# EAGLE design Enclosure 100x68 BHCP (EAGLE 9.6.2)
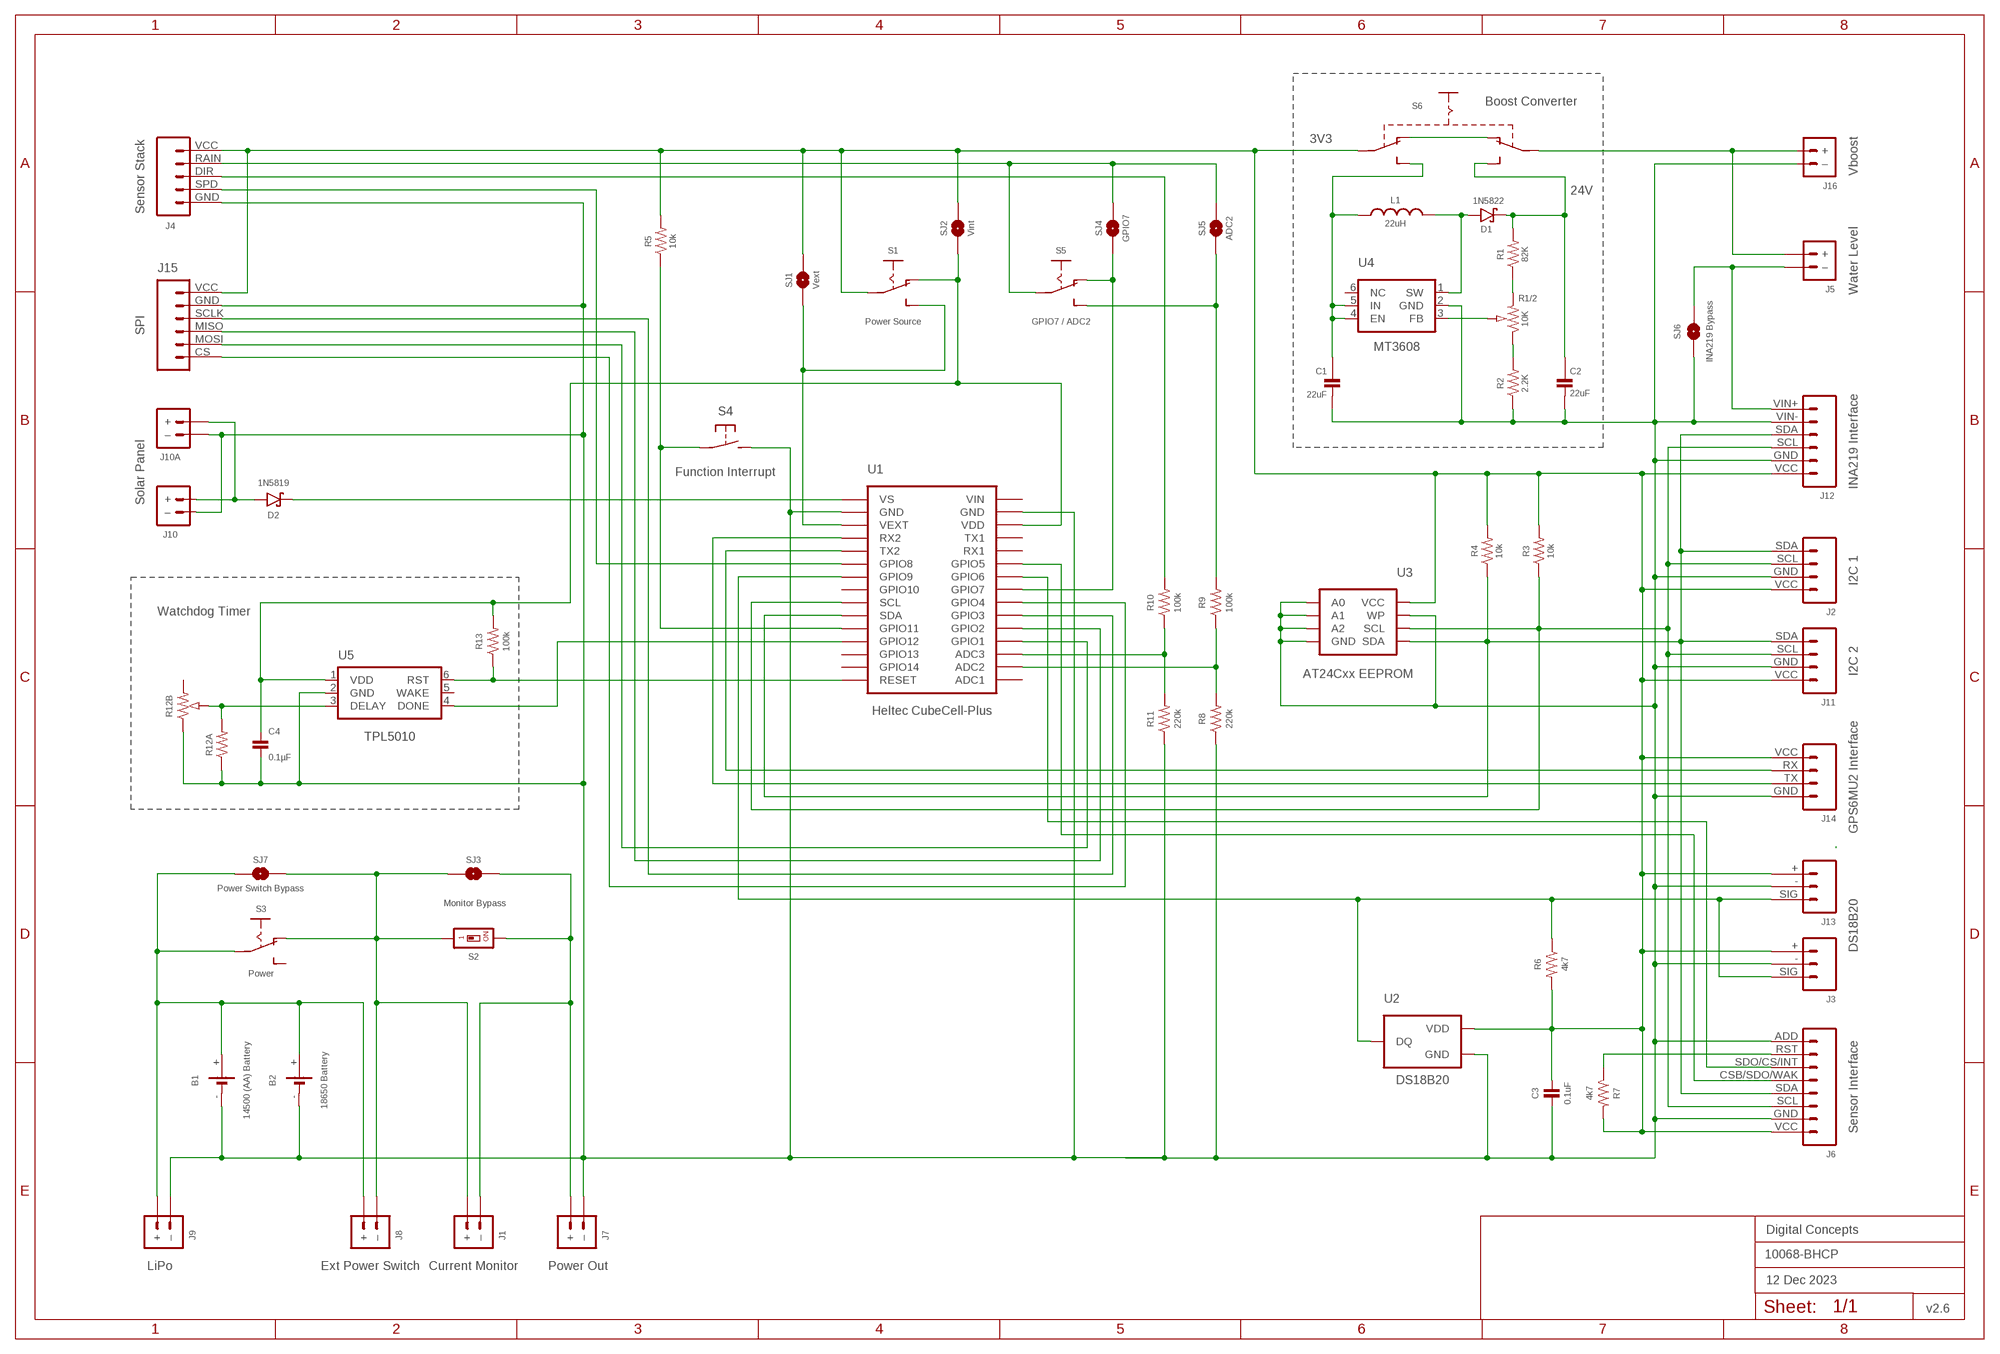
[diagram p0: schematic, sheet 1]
FRAME2 (A3L-LOC): DATE: 12 Dec 2023; OWNER: Digital Concepts; TITLE: 10068-BHCP; VERSION: v2.6

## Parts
B1  14500 (AA) Battery  BATTERY-HOLDER-14500(AA)  [BATTERY-14500]
B2  18650 Battery  BATTERY-HOLDER-18650  [BATTERY-18650]
C1  22uF  CAPACITOR-1206  [C1206]
C2  22uF  CAPACITOR-1206  [C1206]
C3  0.1uF  CAPACITOR-0805  [C0805]
C4  0.1µF  CAPACITOR-0805  [C0805]
D1  1N5822  DIODE-SCHOTTKY-1N5822  [DIODE_SMB]
D2  1N5819  1N5819-SOD-123  [SOD-123]
J1  Current Monitor  JST-PH2.0-2-HORIZONTALJST-PTH-2  [JST-PH2.0-2-HORIZONTAL]
J2  I2C 1  JST-PH2.0-4-VERTICAL-I2C  [JST-PH2.0-4-VERTICAL-I2C]
J3  DS18B20  JST-PH2.0-3-VERTICAL-DS18B20  [JST-PH2.0-3-VERTICAL-SIG]
J4  Sensor Stack  JST-PH2.0-5-DUAL-WEATHER  [JST-PH2.0-5-DUAL-WEATHER]
J5  Water Level  JST-PH2.0-2-DUAL-POWERJST-PTH-2  [JST-PH2.0-2-DUAL-POWER]
J6  Sensor Interface  HEADER-1X8-SENSOR  [CONN_08-SENSOR]
J7  Power Out  JST-GH1.25-2-HORIZONTAL-POWER  [JST-GH1.25-2-HORIZONTAL]
J8  Ext Power Switch  JST-PH2.0-2-DUAL-POWERJST-PTH-2  [JST-PH2.0-2-DUAL-POWER]
J9  LiPo  JST-PH2.0-2-HORIZONTAL-POWERJST-PTH-2  [JST-PH2.0-2-HORIZONTAL-POWER]
J10  Solar Panel  JST-PH2.0-2-VERTICAL  [JST-PH2.0-2-VERTICAL=POWER]
J10A  JST-PH2.0-2-HORIZONTAL-POWERJST-PTH-2  [JST-PH2.0-2-HORIZONTAL-POWER]
J11  I2C 2  JST-PH2.0-I2C-MALE-HORIZONTAL  [JST-PH2.0-4-HORIZONTAL]
J12  INA219 Interface  INA219-I2C-MODULE  [CONN_06-INA219]
J13  JST-PH2.0-3-HORIZONTAL-DS18B20  [JST-PH2.0-DS18B20-HORIZONTAL]
J14  GPS6MU2 Interface  HEADER-1X4-GPS  [CONN_04-GPS]
J15  SPI  JST-PH2.0-6-HORIZONTAL-SPI  [JST-PH2.0-6-HORIZONTAL-SPI]
J16  Vboost  JST-PH2.0-2-VERTICAL  [JST-PH2.0-2-VERTICAL=POWER]
L1  22uH  INDUCTOR-CDRH104R/6D28L5038P  [CDRH104R+6D28]
R1  82K  RESISTORR0805  [R0805]
R1/2  10K  RESISTOR-TRIMM-BAOTER-H-US  [RTRIM64P]
R2  2.2K  RESISTORR0805  [R0805]
R3  10k  RESISTORR0805  [R0805]
R4  10k  RESISTORR0805  [R0805]
R5  10k  RESISTORR0805  [R0805]
R6  4k7  RESISTORR0805  [R0805]
R7  4k7  RESISTORR0805  [R0805]
R8  220k  RESISTORR0805  [R0805]
R9  100k  RESISTORR0805  [R0805]
R10  100k  RESISTORR0805  [R0805]
R11  220k  RESISTORR0805  [R0805]
R12A  RESISTORR0805  [R0805]
R12B  RESISTOR-TRIMM-33-US  [RTRIM3*3]
R13  100k  RESISTORR0805  [R0805]
S1  Power Source  SWITCH-SLIDE-SPDT-SMT  [SWITCH-SPDT-SMT]
S2  Monitor Bypass  SWITCH-DIP-SWS001  [SMD-001]
S3  Power  SWITCH-SLIDE-SPDT-PTH  [SWITCH-SPDT-PTH]
S4  Function Interrupt  SWITCH-MOMENTARY-2-PIN  [SWITCH-2-PAD]
S5  GPIO7 / ADC2  SWITCH-SLIDE-SPDT-SMT  [SWITCH-SPDT-SMT]
S6  SWITCH-SLIDE-DPDT-PTH-S  [SWITCH-DPDT-PTH]
SJ1  Vext  SJ  [SJ]
SJ2  Vint  SJ-V-12  [SJ-VIA-12]
SJ3  Monitor  SJ  [SJ]
SJ4  GPIO7  SJ-V-2  [SJ-VIA-2]
SJ5  ADC2  SJ-V-12  [SJ-VIA-12]
SJ6  INA219 Bypass  SJ  [SJ]
SJ7  Power Switch Bypass  SJ  [SJ]
U1  Heltec CubeCell-Plus  HELTEC-CUBECELL-PLUS-X  [HELTEC-CUBECELL=PLUS-X]
U2  DS18B20  THERMOMETER-DS18B20  [TO-92]
U3  AT24Cxx EEPROM  AT24CXX-EEPROM  [SOP-8]
U4  MT3608  [SOT-23-6]
U5  TPL5010  TPL5010DDCR  [SOT-23-6]

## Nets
GND: B1.- B2.- C1.2 C2.2 C3.2 C4.2 J2.GND J3.- J4.GND J6.ADD J6.GND J7.-(–) J9.-(–) J10.-(–) J10A.-(–) J11.GND J12.GND J12.VIN- J13.- J14.GND J15.GND J16.-(–) R2.1 R8.1 R11.1 R12A.1 R12B.1(A) S4.P$2(S) SJ6.1 U1.GND@14(GND) U1.GND@17(GND) U2.1(GND) U3.P$1(A0) U3.P$2(A1) U3.P$3(A2) U3.P$4(GND) U3.P$7(WP) U4.2(GND) U5.2(GND)
N$1: D2.A J10.+ J10A.+
N$2: R10.1 R11.2 U1.ADC3
N$3: J1.2(–) J7.+ S2.2 SJ3.1
N$4: B1.+ B2.+ J8.+ J9.+ S3.2(P) SJ7.2
N$5: D2.C U1.VS
N$6: D1.A L1.1 U4.1(SW)
N$7: J4.DIR R10.2
N$8: J2.SCL J6.SCL J11.SCL J12.SCL R3.1 U1.SCL U3.P$6(SCL)
N$9: J6.RST R7.1
N$10: J6.CSB/SDO/WAK U1.GPIO5
N$11: J2.SDA J6.SDA J11.SDA J12.SDA R4.1 U1.SDA U3.P$5(SDA)
N$12: J4.SPD U1.GPIO8
N$13: S1.3(S) SJ1.1 U1.VEXT
N$14: J14.RX U1.TX2
N$15: J5.-(–) J12.VIN+ SJ6.2
N$16: J14.TX U1.RX2
N$18: R12A.2 R12B.2(S) U5.3(DELAY)
N$19: J6.SDO/CS/INT U1.GPIO6
N$20: J5.+ J16.+ S6.P$2(P1)
N$21: J1.1(+) J8.-(–) S2.1 S3.1(O) SJ3.2 SJ7.1
N$22: R1/2.2(S) U4.3(FB)
N$23: R1/2.1(A) R2.2
N$24: J3.SIG J13.SIG R6.1 U1.GPIO9 U2.2(DQ)
N$25: C1.1 L1.2 S6.P$6(S2) U4.4(EN) U4.5(IN)
N$26: S6.P$1(O1) S6.P$4(O2)
N$27: R5.1 S4.P$1(P) U1.GPIO11
N$28: C2.1 D1.C R1.2 S6.P$3(S1)
N$29: J15.MOSI U1.GPIO1
N$30: J15.MISO U1.GPIO2
N$31: R9.2 S5.3(S) SJ5.1 SJ5.1@V
N$32: J4.RAIN S5.2(P) SJ4.2 SJ4.2@V SJ5.2 SJ5.2@V
N$33: R8.2 R9.1 U1.ADC2
N$34: R13.1 U1.RST(RESET) U5.6(RST)
N$35: J15.SCLK U1.GPIO3
N$36: J15.CS U1.GPIO4
N$37: U1.GPIO12 U5.4(DONE)
N$38: R1.1 R1/2.3(E)
N$39: C4.1 R13.2 S1.1(O) SJ2.1 SJ2.1@V U1.VDD U5.1(VDD)
N$40: S5.1(O) SJ4.1 U1.GPIO7
VEXT: C3.1 J2.VCC J3.+ J4.VCC J6.VCC J11.VCC J12.VCC J13.+ J14.VCC J15.VCC R3.2 R4.2 R5.2 R6.2 R7.2 S1.2(P) S6.P$5(P2) SJ1.2 SJ2.2 SJ2.2@V U2.3(VDD) U3.P$8(VCC)
Unconnected: R12B.3(E) S3.3(S) U1.ADC1 U1.GPIO10 U1.GPIO13 U1.GPIO14 U1.RX1 U1.TX1 U4.6(NC) U5.5(WAKE)

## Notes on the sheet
- Boost Converter
- 3V3
- 24V
- Watchdog Timer

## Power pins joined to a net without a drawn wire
VIN: U1.VIN

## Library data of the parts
B1 = digitalconcepts:BATTERY-HOLDER-14500(AA): 14500 (AA) battery holder
B2 = digitalconcepts:BATTERY-HOLDER-18650: 18650 Battery Holder
C1 C2 = digitalconcepts:CAPACITOR-1206: 1206 Capacitor
C3 C4 = digitalconcepts:CAPACITOR-0805: 0805 Capacitor
D1 = digitalconcepts:DIODE-SCHOTTKY-1N5822: 1N5822 Schottky Diode SMB
D2 = digitalconcepts:1N5819-SOD-123: 1N5819 Schottky Diode SOD-123
J1 = digitalconcepts:JST-PH2.0-2-HORIZONTAL: PH2.0 2P Right Angle PCB Connector; PROD_ID: CONN-09863; SKU: PRT-09914
J2 = digitalconcepts:JST-PH2.0-4-VERTICAL-I2C: PH2.0 4P I2C Vertical Connector
J3 = digitalconcepts:JST-PH2.0-3-VERTICAL-DS18B20: DS18B20 PH2.0 Vertical PCB Connector
J4 = digitalconcepts:JST-PH2.0-5-DUAL-WEATHER: PH2.0 5P Dual Connector
J5 J8 = digitalconcepts:JST-PH2.0-2-DUAL-POWER: JST PH2.0 2P PTH Dual-Side Connector (Power); PROD_ID: CONN-09863; SKU: PRT-09914
J6 = digitalconcepts:HEADER-1X8-SENSOR: IoT Sensors 1x8 Pin Header for 'Sandwich' IoT Sensors
J7 = digitalconcepts:JST-GH1.25-2-HORIZONTAL-POWER: JST GH1.25 2P PTH Connector (Power)
J9 J10A = digitalconcepts:JST-PH2.0-2-HORIZONTAL-POWER: PH2.0 2P Right Angle PCB Connector; PROD_ID: CONN-09863; SKU: PRT-09914
J10 J16 = digitalconcepts:JST-PH2.0-2-VERTICAL: PH2.0 2P PCB Connector
J11 = digitalconcepts:JST-PH2.0-I2C-MALE-HORIZONTAL: PH2.0 4P (I2C) Right Angle PCB Connector
J12 = digitalconcepts:INA219-I2C-MODULE: INA219 I2C Module
J13 = digitalconcepts:JST-PH2.0-3-HORIZONTAL-DS18B20: DS18B20 PH2.0 Right Angle PCB Connector
J14 = digitalconcepts:HEADER-1X4-GPS: NEO GPS 4-Pin Header
J15 = digitalconcepts:JST-PH2.0-6-HORIZONTAL-SPI: PH2.0 6P Horizontal Connector—SPI
L1 = digitalconcepts:INDUCTOR-CDRH104R/6D28: Inductor; SPICEPREFIX: L
R1-R11 R12A R13 = digitalconcepts:RESISTOR: Resistor; SPICEPREFIX: R
R1/2 = digitalconcepts:RESISTOR-TRIMM-BAOTER-H-US: Trimm Resistor - Horizontal BAOTER
R12B = digitalconcepts:RESISTOR-TRIMM-3*3-US: Trimm Resistor - 3*3 SMD
S1 S5 = digitalconcepts:SWITCH-SLIDE-SPDT-SMT: Mini Sliding Switch SPDT SMT
S2 = digitalconcepts:SWITCH-DIP-SWS001: SMD Dip Switch 1 pol.
S3 = digitalconcepts:SWITCH-SLIDE-SPDT-PTH: Mini Sliding Switch SPDT PTH
S4 = digitalconcepts:SWITCH-MOMENTARY-2-PIN: 2 Pin Momentary Switch
S6 = digitalconcepts:SWITCH-SLIDE-DPDT-PTH-S: Switch DPDT PTH-S
SJ1 SJ3 SJ6 SJ7 = digitalconcepts:SJ: Solder Jumper
SJ2 SJ5 = digitalconcepts:SJ-V-12: Solder Jumper with Pad Vias
SJ4 = digitalconcepts:SJ-V-2: Solder Jumper with Pad Vias
U1 = digitalconcepts:HELTEC-CUBECELL-PLUS-X: Heltec CubeCell Dev-Board Plus Excluding internal pins
U2 = digitalconcepts:THERMOMETER-DS18B20: Digital Thermometer -55C-125C TO92-3; AVAILABILITY: Bad; DESCRIPTION: Temperature Sensor Digital, Local -55°C ~ 125°C 12 b 8-uMAX; MF: Maxim Integrated; MP: DS18B20; PACKAGE: TO-92 Maxim Integrated; PRICE: None
U3 = digitalconcepts:AT24CXX-EEPROM: AT24Cxx EEPROM SOP-8
U4 = digitalconcepts:MT3608: MT3608 DC-DC Step-Up Voltage Converter
U5 = digitalconcepts:TPL5010DDCR: TPL5010 Nano-Power System Timer with Watchdog

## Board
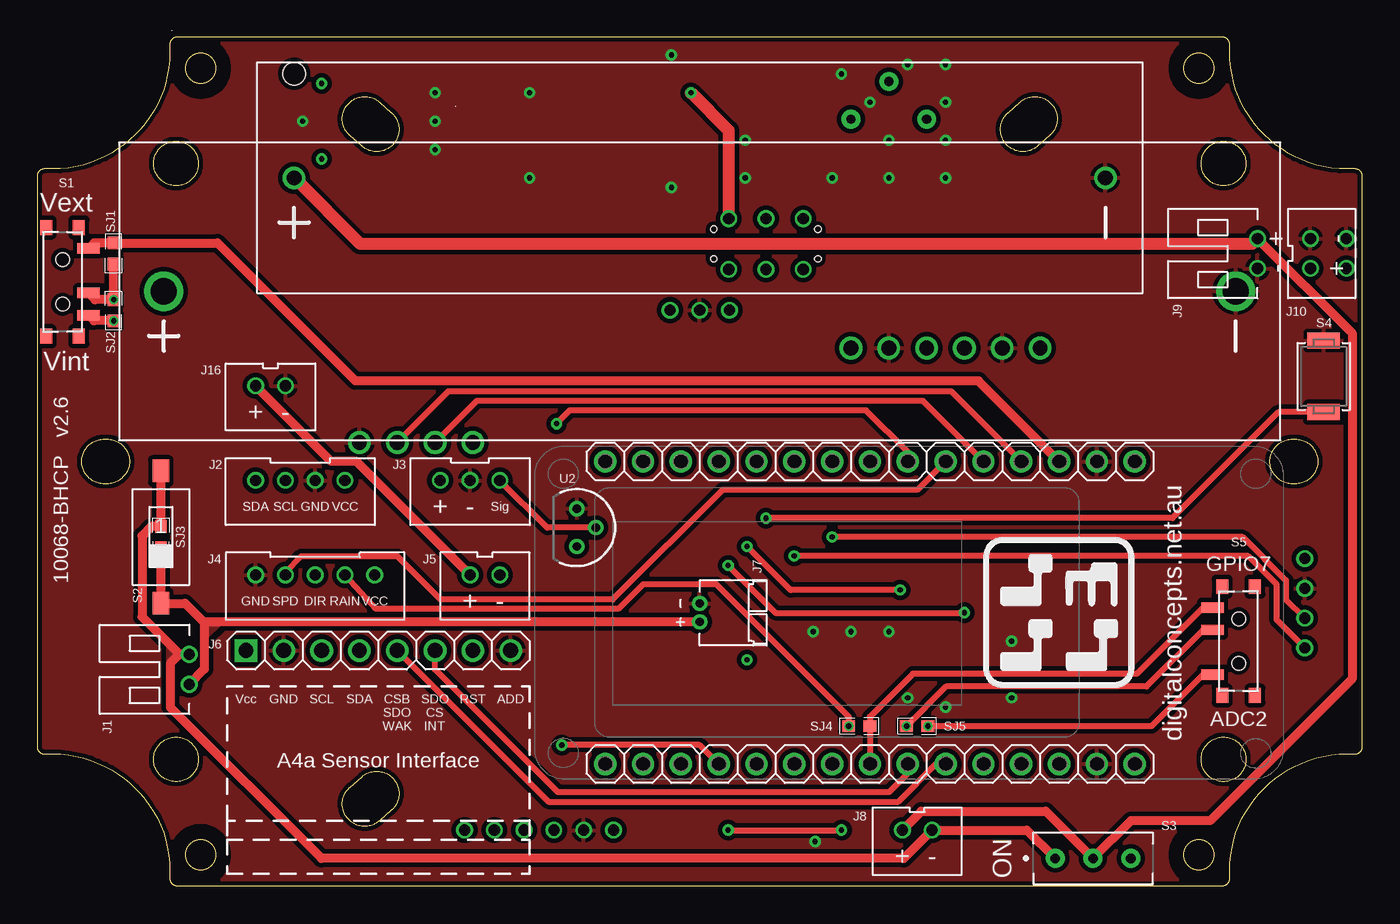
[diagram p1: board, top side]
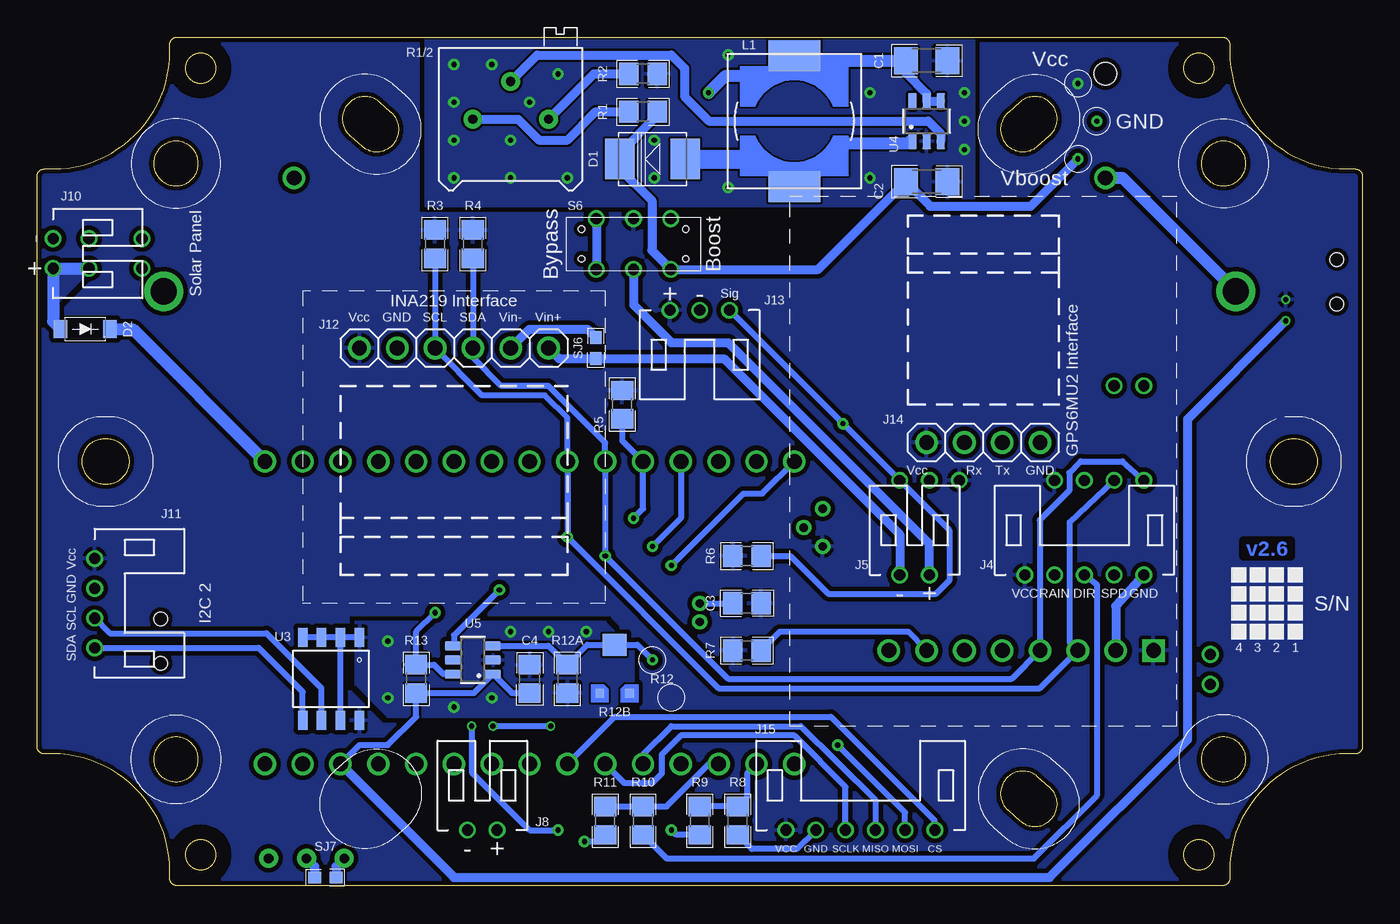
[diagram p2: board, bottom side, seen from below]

Size 89 x 57 mm. Coordinates in mm from the lower left corner, seen from the top.
Outline: 1134 segments
Outline: circle at 10.97,2.08 radius 1.02
Outline: circle at 10.97,54.92 radius 1.02
Outline: circle at 78.03,54.92 radius 1.02
Outline: circle at 78.03,2.08 radius 1.02
Copper layers (1*16): Top 0.035mm / dielectric 1.5mm / Bottom 0.035mm
Design rules "default *": minimum track width 6mil, minimum drill 0.35mm, track to track 6mil, track to pad 6mil, pad to pad 6mil, via to via 6mil, smd to smd 6mil, copper to edge 6mil, drill to drill 6mil, minimum pad ring 1mil, minimum via ring 8mil, stop-mask expansion 4mil, vias tented up to drill 0mil, thermal gap 10mil

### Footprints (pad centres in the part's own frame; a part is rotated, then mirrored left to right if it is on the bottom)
BATTERY-14500 = drill 1: + -27.25,0; - 27.25,0 | hole 1.524: -27.25,7
BATTERY-18650 = drill 1.75: + -36,0; - 36,0
C1206 = smd 1.6 x 1.8: 1 -1.4,0; 2 1.4,0
C0805 = smd 1.3 x 1.5: 1 -0.95,0; 2 0.95,0
DIODE_SMB = smd 2 x 2.7: A 2.2,0; C -2.2,0
SOD-123 = smd 0.91 x 1.22: A -1.65,0; C 1.65,0
JST-PH2.0-2-HORIZONTAL = drill 0.75: 1 1,0; 2 -1,0
JST-PH2.0-4-VERTICAL-I2C = drill 0.75: GND 1,0; SCL -1,0; SDA -3,0; VCC 3,0
JST-PH2.0-3-VERTICAL-SIG = drill 0.75: + -2,0; - 0,0; SIG 2,0
JST-PH2.0-5-DUAL-WEATHER = drill 0.75: DIR 0,0; GND 4,0; RAIN -2,0; SPD 2,0; VCC -4,0
JST-PH2.0-2-DUAL-POWER = drill 0.75: + 1,0; - -1,0
CONN_08-SENSOR = drill 1 pad 1.524: ADD 17.78,0; CSB/SDO/WAK 10.16,0; GND 2.54,0; RST 15.24,0; SCL 5.08,0; SDA 7.62,0; SDO/CS/INT 12.7,0 | drill 1 pad 1.524 square: VCC 0,0
JST-GH1.25-2-HORIZONTAL = drill 0.55 pad 1.016: + -0.625,0; - 0.625,0
JST-PH2.0-2-HORIZONTAL-POWER = drill 0.75: + 1,0; - -1,0
JST-PH2.0-2-VERTICAL=POWER = drill 0.75: + -1,0; - 1,0
JST-PH2.0-4-HORIZONTAL = drill 0.75: GND -1,0; SCL 1,0; SDA 3,0; VCC -3,0
CONN_06-INA219 = drill 1 pad 1.524: GND 2.54,0; SCL 5.08,0; SDA 7.62,0; VCC 0,0; VIN+ 12.7,0; VIN- 10.16,0
JST-PH2.0-DS18B20-HORIZONTAL = drill 0.75: + 2,0; - 0,0; SIG -2,0
CONN_04-GPS = drill 1 pad 1.524: GND 0,0; RX 5.08,0; TX 2.54,0; VCC 7.62,0
JST-PH2.0-6-HORIZONTAL-SPI = drill 0.75: CS 5,0; GND -3,0; MISO 1,0; MOSI 3,0; SCLK -1,0; VCC -5,0
CDRH104R+6D28 = smd 2.1 x 3.5: 1 -4.4,0; 2 4.4,0
R0805 = smd 1.3 x 1.5: 1 -0.95,0; 2 0.95,0
RTRIM64P = drill 0.61 pad 1.27: 1 0,-2.54; 2 2.54,0; 3 0,2.54
RTRIM3*3 = smd 0.6 x 0.6: 1 -1,-1.6; 3 1,-1.6 | smd 1.6 x 1.5: 2 0,1.65
SWITCH-SPDT-SMT = smd 0.7 x 1.5: 1 2.25,1.75; 2 0.75,1.75; 3 -2.25,1.75 | smd 1 x 0.8: GND@1 3.65,-1.1; GND@2 3.65,1.1; GND@3 -3.65,1.1; GND@4 -3.65,-1.1 | hole 0.9: -1.5,0; 1.5,0
SMD-001 = smd 1.1 x 1.5: 1 0,-4.45; 2 0,4.45
SWITCH-SPDT-PTH = drill 0.65 pad 1.27: 1 -2.54,0; 2 0,0; 3 2.54,0
SWITCH-2-PAD = smd 1.067 x 2.184: P$1 -2.4,0; P$2 2.4,0
SWITCH-DPDT-PTH = drill 0.75: P$1 -1.7,2.5; P$2 -1.7,0; P$3 -1.7,-2.5; P$4 1.7,2.5; P$5 1.7,0; P$6 1.7,-2.5 | hole 0.42: 1,3.5; -1,3.5; 1,-3.5; -1,-3.5
SJ = smd 0.864 x 0.762: 1 -0.711,0; 2 0.711,0
SJ-VIA-12 = smd 0.864 x 0.762: 1 -0.711,0; 2 0.711,0 | drill 0.35 pad 0.61: 1@V -0.711,0; 2@V 0.711,0
SJ-VIA-2 = smd 0.864 x 0.762: 1 -0.711,0; 2 0.711,0 | drill 0.35 pad 0.61: 2@V 0.711,0
HELTEC-CUBECELL=PLUS-X = drill 1: ADC1 0,0; ADC2 0,2.54; ADC3 0,5.08; GND@14 0,33.02; GND@17 -20.32,33.02; GPIO1 0,7.62; GPIO2 0,10.16; GPIO3 0,12.7; GPIO4 0,15.24; GPIO5 0,22.86; GPIO6 0,20.32; GPIO7 0,17.78; GPIO8 -20.32,22.86; GPIO9 -20.32,20.32; GPIO10 -20.32,17.78; GPIO11 -20.32,10.16; GPIO12 -20.32,7.62; GPIO13 -20.32,5.08; GPIO14 -20.32,2.54; RST -20.32,0; RX1 0,25.4; RX2 -20.32,27.94; SCL -20.32,15.24; SDA -20.32,12.7; TX1 0,27.94; TX2 -20.32,25.4; VDD 0,30.48; VEXT -20.32,30.48; VIN 0,35.56; VS -20.32,35.56
TO-92 = drill 0.55 pad 1.016: 1 -1.27,0; 2 0,1.27; 3 1.27,0
SOP-8 = smd 0.635 x 1.27: P$1 -1.905,-2.794; P$2 -0.635,-2.794; P$3 0.635,-2.794; P$4 1.905,-2.794; P$5 1.905,2.794; P$6 0.635,2.794; P$7 -0.635,2.794; P$8 -1.905,2.794
SOT-23-6 = smd 1.1 x 0.6: 1 -1.35,0.95; 2 -1.35,0; 3 -1.35,-0.95; 4 1.35,-0.95; 5 1.35,0; 6 1.35,0.95

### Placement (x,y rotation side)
B1  44.5,47.55 0 top
B2  44.5,39.93 0 top
C1  29.26,55.42 0 bottom
C2  29.26,47.3 0 bottom
C3  41.32,18.97 180 bottom
C4  55.93,13.89 90 bottom
D1  47.67,48.82 0 bottom
D2  85.77,37.39 0 bottom
J1  10.21,14.53 90 top
J2  17.67,27.23 0 top
J3  29.07,27.23 0 top
J4  18.67,20.88 0 bottom
J5  30.07,20.88 0 bottom
J6  14.02,15.8 0 top
J7  44.5,18.34 90 top
J8  59.1,3.73 0 bottom
J9  81.96,42.47 90 top
J10  85.52,42.47 90 top
J10A  87.93,42.47 270 bottom
J11  85.14,18.97 270 bottom
J12  67.36,36.12 0 bottom
J13  44.5,38.66 180 bottom
J14  21.64,29.77 180 bottom
J15  33.7,3.73 0 bottom
J16  15.67,33.58 0 top
L1  38.15,51.36 90 bottom
R1  48.31,51.99 0 bottom
R1/2  57.2,51.49 90 bottom
R2  48.31,54.53 180 bottom
R3  62.28,43.1 90 bottom
R4  59.74,43.1 90 bottom
R5  49.71,32.31 90 bottom
R6  41.32,22.15 180 bottom
R7  41.32,15.8 180 bottom
R8  41.96,4.37 90 bottom
R9  44.5,4.37 270 bottom
R10  48.31,4.37 270 bottom
R11  50.85,4.37 90 bottom
R12A  53.39,13.89 90 bottom
R12B  50.21,14.53 0 bottom
R13  63.55,13.89 270 bottom
S1  1.7,40.56 270 top
S2  8.3,23.42 180 top
S3  70.92,1.83 0 top
S4  86.41,34.21 90 top
S5  80.69,16.43 90 top
S6  48.94,43.1 90 bottom
SJ1  5.13,42.47 270 top
SJ2  5.13,38.66 90 top
SJ3  8.3,23.42 90 top
SJ4  55.22,10.72 180 top
SJ5  59.1,10.72 180 top
SJ6  51.48,36.12 270 bottom
SJ7  69.65,0.56 180 bottom
U1  38.15,8.18 270 top
U2  36.24,24.05 270 top
U3  69.26,13.89 180 bottom
U4  29.26,51.36 90 bottom
U5  59.74,15.16 180 bottom

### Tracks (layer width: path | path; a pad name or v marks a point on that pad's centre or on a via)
$X
  cutout Bottom: 10.97,56.95 arc180 10.97,52.88 arc180
$X1
  cutout Bottom: 78.03,56.95 arc180 78.03,52.88 arc180
$X2
  cutout Top: 78.03,4.12 arc180 78.03,0.05 arc180
$X3
  cutout Top: 10.97,4.12 arc180 10.97,0.05 arc180
$X4
  cutout Top: 10.97,56.95 arc180 10.97,52.88 arc180
$X5
  cutout Top: 78.03,56.95 arc180 78.03,52.88 arc180
$X6
  cutout Bottom: 78.03,4.12 arc180 78.03,0.05 arc180
$X7
  cutout Bottom: 10.97,4.12 arc180 10.97,0.05 arc180
GND  (via drill 0.35)
  Bottom 0.406: R11.1 51.3,2.97 v52.25,2.97 | J7.- C3.2 | U3.P$7 U3.P$2 | U3.P$1 U3.P$2 | U3.P$2 U3.P$3 U3.P$4 | R12B.1 50.86,12.93 | J15.GND 37.97,2.46 41,2.46 R8.1
  Bottom 0.61: J4.GND 16.56,18.78 J6.GND | J12.VIN- 55.93,37.39 52.04,37.39 SJ6.1
  other vias: 26.72,53.26 58.47,55.17 54.02,54.53 47.55,50.09 47.55,47.55 53.39,47.55 57.2,47.55 57.2,50.09 61.01,47.55 61.01,50.09 61.01,55.17 26.72,51.36 55.93,52.63 61.01,52.63 42.59,46.91 42.59,55.8 33.07,53.26 33.07,47.55 26.72,49.45 17.83,51.36 52.12,17.07 54.66,17.07 57.2,17.07 65.45,16.43 65.45,12.62 61.01,11.99 58.47,12.62
  pour Top (isolate 0.305, rank 2): -1.65,58.87 -1.65,-1.92 90.59,-1.92 90.59,58.87
  pour Bottom: 26.08,57.07 26.08,45.64 62.91,45.64 62.91,57.07
  pour Bottom: 67.61,17.7 67.61,13.51 65.45,11.35 50.85,11.35 48.94,13.26 48.94,15.8 50.85,17.7
N$1
  Bottom 0.813: D2.A 87.93,37.9 J10A.+ J10.+
  pour Bottom (no thermals): 85.77,41.47 87.93,41.47 87.93,39.31
N$2
  Bottom 0.406: R11.2 R10.1 46.72,5.32 43.86,8.18 U1.ADC3
N$3
  Top 0.61: SJ3.1 S2.2 9.93,18.97 11.23,17.67 | 11.23,17.67 11.23,14.55 J1.2 | 11.23,17.67 11.27,17.71 J7.+
  pour Top: 11.23,17.71 11.23,16.43 12.51,17.71
N$4
  Top 0.61: J9.+ 88.31,37.12 88.31,13.89 78.79,4.37 73.46,4.37 S3.2 67.74,5 59.37,5 J8.+
  Top 0.813: J9.+ 81.6,43.1 21.69,43.1 B1.+
  Bottom 0.61: S3.2 70.36,1.27 SJ7.2
  Bottom 0.813: B1.+ 16.12,47.55 B2.+
N$5
  Bottom 0.813: D2.C 82.6,37.39 U1.VS
N$6
  Bottom 0.152: U4.1 30.4,50.01
  Bottom 0.406: 40.5,48.82 38.64,46.96 L1.1 37.96,46.96 35.04,49.88
  Bottom 0.813: 35.04,49.88 30.53,49.88 30.4,50.01
  Bottom 1.27: D1.A 40.5,48.82
N$7
  Bottom 0.406: J4.DIR 17.83,20.24 17.83,6.05 22.05,1.83 46.72,1.83 R10.2
N$8  (via drill 0.35)
  Top 0.406: J11.SCL 83.87,19.24 83.87,20.51 80.96,23.42 v53.39,23.42
  Bottom 0.406: J2.SCL 19.66,24.41 19.66,16.36 J6.SCL 21.64,13.26 43.23,13.26 v53.39,23.42 U1.SCL 53.39,31.42 54.91,32.94 59.1,32.94 J12.SCL R3.1 | U3.P$6 69.9,13.26 73.6,16.96 84.12,16.96 J11.SCL
N$9
  Bottom 0.406: R7.1 39.1,17.07 30.53,17.07 J6.RST
N$10
  Top 0.406: J6.CSB/SDO/WAK 34.34,5.64 57.83,5.64 60.37,8.18 U1.GPIO5
N$11  (via drill 0.35)
  Top 0.406: J11.SDA 83.23,17.88 83.23,20.26 81.34,22.15 v50.85,22.15
  Bottom 0.406: J2.SDA 16.1,28.5 18.92,28.5 19.68,27.73 19.68,26.54 21.66,24.56 21.66,15.82 J6.SDA 23.54,13.89 42.59,13.89 v50.85,22.15 U1.SDA 50.85,29.77 54.66,33.58 57.83,33.58 59.74,35.48 J12.SDA R4.1 | J11.SDA 74.14,15.97 71.17,13.01 U3.P$5
N$12
  Top 0.406: U1.GPIO8 59.1,26.59 46.02,26.59 38.66,19.23 27.1,19.23 24.18,22.15 17.73,22.15 16.67,21.08 J4.SPD
N$13
  Top 0.61: U1.VEXT 63.22,33.91 21.39,33.91 12.11,43.18 SJ1.1 3.82,43.18 S1.3
N$14
  Top 0.406: J14.RX 29.51,32.56 59.49,32.56 U1.TX2
N$15
  Bottom 0.61: J5.- 31.07,23.59 42.88,35.41 SJ6.2 53.95,35.41 J12.VIN+
N$16
  Top 0.406: J14.TX 27.61,33.2 61.39,33.2 U1.RX2
N$18  (via drill 0.35)
  Bottom 0.406: U5.3 54.66,16.11 R12A.2 52.05,16.18 R12B.2 48.69,16.18 v47.67,15.16
N$19
  Top 0.406: J6.SDO/CS/INT 26.72,14.53 34.97,6.27 57.2,6.27 58.47,7.54 U1.GPIO6
N$20
  Top 0.61: J5.+ 21.45,28.5 19.75,28.5 J16.+
  Bottom 0.61: S6.P$2 48.94,39.02 46.4,36.48 42.59,36.48 29.07,22.96 J5.+
N$21
  Top 0.61: S2.1 SJ3.2 7.67,24.13 7.03,23.5 7.03,18.07 9.57,15.53 J1.1 9.55,15.53 8.94,14.92 8.94,11.99 19.1,1.83 58.2,1.83 J8.- 66.47,3.73 S3.1
  Bottom 0.61: S3.1 68.93,1.27 SJ7.1
  pour Top: 9.55,15.55 8.94,16.16 8.94,14.94
N$22
  Bottom 0.61: U4.3 28.31,50.51 29.16,51.36 43.86,51.36 45.52,53.01 45.52,54.92 46.4,55.8 55.42,55.8 R1/2.2
N$23
  Bottom 0.61: R1/2.1 51.61,54.53 R2.2
N$24  (via drill 0.35)
  Top 0.406: U1.GPIO9 58.47,29.13 55.68,31.93 35.77,31.93 v34.88,31.04 | U2.2 34.24,24.05 J3.SIG
  Bottom 0.406: R6.1 38.4,22.15 35.86,19.61 28.62,19.61 27.74,20.5 27.74,23.9 J3.SIG v34.88,31.04 J13.SIG
N$25  (via drill 0.35)
  Top 0.813: v43.9,53.26 46.44,50.72 S6.P$6
  Bottom 0.61: C1.1 30.66,54.61 29.26,53.21 U4.5 U4.4
  Bottom 0.813: C1.1 37.68,55.42 L1.2 38.53,55.76 39.88,54.41 42.76,54.41 v43.9,53.26
N$26
  Bottom 0.61: S6.P$4 S6.P$1
N$27  (via drill 0.35)
  Top 0.406: S4.P$1 83.37,31.81 76.25,24.69 v48.94,24.69
  Bottom 0.406: v48.94,24.69 48.31,25.32 U1.GPIO11 49.71,29.9 R5.1
N$28  (via drill 0.35)
  Bottom 0.61: v19.1,48.82 22.27,45.64 29.01,45.64 C2.1 36.55,41.4 S6.P$3 47.71,42.67 47.71,46.02 49.87,48.18 D1.C 50,48.95 50,49.07 47.36,51.71 R1.2
N$29  (via drill 0.35)
  Top 0.406: U1.GPIO1 44.5,9.45 v35.23,9.45
  Bottom 0.406: v35.23,9.45 30.7,4.92 J15.MOSI
N$30
  Bottom 0.406: J15.MISO 32.7,5.76 37.71,10.72 46.4,10.72 48.31,8.81 U1.GPIO2
N$31  (via drill 0.35)
  Top 0.406: S5.3 78.31,14.18 74.84,10.72 SJ5.1@V | v46.4,3.73 v54.02,3.73
  Bottom 0.406: SJ5.1@V 59.82,7.62 55.93,3.73 v54.02,3.73 | R9.2 46.09,3.42 v46.4,3.73
N$32
  Top 0.406: J4.RAIN 22.75,18.59 39.04,18.59 40.69,20.24 45.62,20.24 54.51,11.35 SJ4.2@V | S5.2 78.31,17.18 74.5,13.37 61.05,13.37 SJ5.2
  Bottom 0.406: SJ4.2@V SJ5.2
N$33
  Bottom 0.406: R9.1 R8.2 41.32,5.95 41.32,7.54 U1.ADC2
N$34  (via drill 0.35)
  Top 0.406: v46.4,21.51 49.58,18.34 v62.28,18.34
  Bottom 0.406: U5.6 61.72,14.21 62.36,14.85 64.18,14.85 64.17,14.84 R13.1 63.55,17.07 v62.28,18.34 | U1.RST 40.31,26.34 41.58,26.34 v46.4,21.51
N$35
  Bottom 0.406: J15.SCLK 34.7,6.64 38.15,10.08 45.77,10.08 47.04,8.81 47.04,7.54 47.67,6.91 49.58,6.91 U1.GPIO3
N$36
  Bottom 0.406: J15.CS 28.7,4.37 35.69,11.35 50.21,11.35 U1.GPIO4
N$37  (via drill 0.35)
  Top 0.406: v47.67,22.78 50.6,19.86 v57.96,19.86
  Bottom 0.406: U5.4 61.01,16.19 61.01,16.82 v57.96,19.86 | U1.GPIO12 45.77,24.69 v47.67,22.78
N$38
  Bottom 0.61: R1/2.3 56.69,51.49 55.29,50.09 53.39,50.09 51.48,51.99 R1.1
N$39
  Top 0.61: SJ2.1@V 3.82,37.95 S1.1
  Bottom 0.406: C4.1 57.12,12.94 U5.1 59.66,12.94 R13.2 63.55,11.35 65.45,9.45 67.36,9.45 U1.VDD
  Bottom 0.61: U1.VDD 61.01,0.56 21,0.56 11.73,9.83 11.73,31.34 SJ2.1@V
N$40
  Top 0.406: U1.GPIO7 SJ4.1 55.93,11.35 58.81,14.24 73.86,14.24 78.31,18.68 S5.1
VEXT  (via drill 0.35)
  Top 0.61: S1.2 3.89,39.37 SJ2.2@V SJ1.2
  other vias: 19.1,53.9
  pour Bottom (isolate 0.305, rank 2): -0.65,57.87 -0.65,-0.92 89.59,-0.92 89.59,57.87

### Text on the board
Bottom: v2.6
tPlace: 10068-BHCP v2.6 | digitalconcepts.net.au | Vcc | GND | SCL | SDA | RST | ADD | CSB / SDO / WAK | SDO / CS / INT
bPlace: Vin+ | Vin- | SDA | SCL | GND | Vcc | GND | Tx | Rx | Vcc | S/N | 1 | 2 | 3 | 4
tNames: Vext | Vint | GPIO7 | ADC2 | A4a Sensor Interface | ON
bNames: Vcc | GND | Vboost | J10 | Boost | Bypass | Solar Panel | Vcc | J4 | J5 | GND | SCL | SDA | R12 | J8
tValues: INT | Water Level
bValues: Wind/Rain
